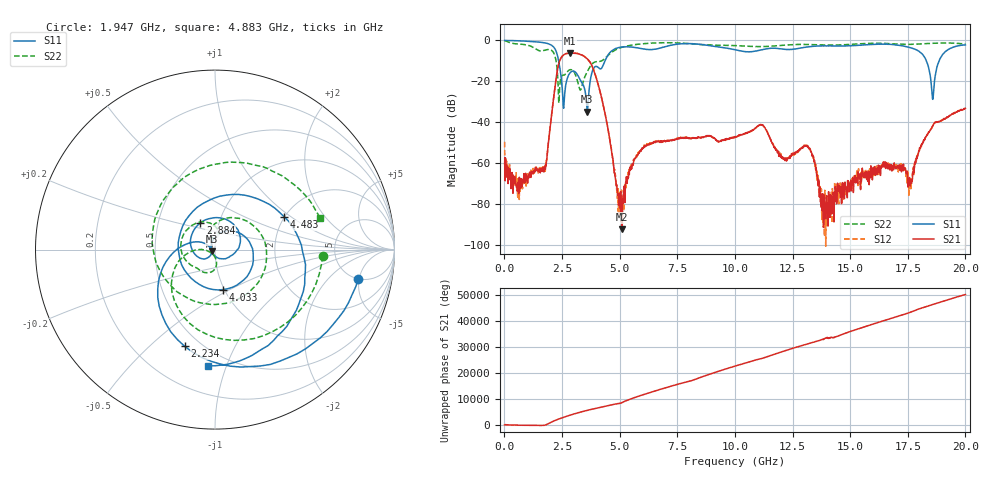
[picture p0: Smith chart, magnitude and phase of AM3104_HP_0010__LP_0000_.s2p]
!Created with skrf (http://scikit-rf.org).
# Hz S RI R 50.0
!freq ReS11 ImS11 ReS21 ImS21 ReS12 ImS12 ReS22 ImS22
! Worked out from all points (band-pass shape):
!   1601 points, 10 MHz to 20 GHz, reference 50 ohm
!   highest |S21| = -6.12 dB at 2.846 GHz (marker M1); lowest = -92.2 dB at 5.095 GHz (marker M2)
!   |S21| within 3 dB of the highest: 2.43 GHz to 3.607 GHz (1.177 GHz wide, 39 % of centre)
!   lowest |S11| = -34.8 dB at 3.596 GHz (marker M3), VSWR 1.04, Z = 48.4 - j0.872 ohm
!   |S11| at or under -10 dB: 2.354 GHz to 4.364 GHz (2.01 GHz wide, 59.8 % of centre); 18.31 GHz to 18.86 GHz (548.4 MHz wide, 2.95 % of centre)
!   |S22| runs from -30.5 to -0.2 dB; largest |S21 - S12| = 0.0045
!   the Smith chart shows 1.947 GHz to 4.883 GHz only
!   S11 on the Smith chart (normalised r, x): 1.947 GHz: 5.01, -4.88; 2.234 GHz: 0.41, -0.65; 2.884 GHz: 0.81, +0.25; 4.033 GHz: 0.99, -0.46; 4.483 GHz: 2.00, +0.88; 4.883 GHz: 0.39, -0.86
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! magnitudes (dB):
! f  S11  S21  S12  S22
! 10 MHz  0.0  -60.3  -49.5  -0.2
! 672.2 MHz  -0.2  -69.4  -73.0  -1.8
! 1.709 GHz  -1.1  -63.1  -63.0  -4.9
! 1.947 GHz  -1.8  -46.1  -46.3  -4.4
! 2.234 GHz  -5.0  -19.4  -19.4  -9.4
! 2.559 GHz  -32.6  -7.1  -7.1  -16.9
! 2.846 GHz  -15.9  -6.1  -6.1  -14.3
! 2.884 GHz  -15.4  -6.2  -6.1  -14.2
! 3.346 GHz  -20.4  -7.0  -7.1  -23.0
! 3.596 GHz  -34.8  -9.0  -8.9  -15.2
! 4.033 GHz  -12.9  -20.0  -19.9  -10.3
! 4.483 GHz  -7.4  -42.5  -42.6  -7.5
! 4.883 GHz  -3.8  -71.2  -74.8  -4.3
! 5.095 GHz  -3.3  -92.2  -84.7  -3.3
! 6.682 GHz  -3.9  -49.2  -48.9  -1.2
! 10.01 GHz  -4.5  -47.2  -47.2  -2.5
! 13.34 GHz  -2.9  -55.3  -55.8  -2.0
! 13.93 GHz  -2.7  -87.0  -79.3  -2.2
! 16.68 GHz  -1.8  -60.5  -61.0  -1.5
! 17.6 GHz  -3.5  -71.1  -69.0  -1.9
! 18.59 GHz  -28.8  -41.4  -41.6  -1.4
! 20 GHz  -2.2  -33.2  -33.3  -1.7
